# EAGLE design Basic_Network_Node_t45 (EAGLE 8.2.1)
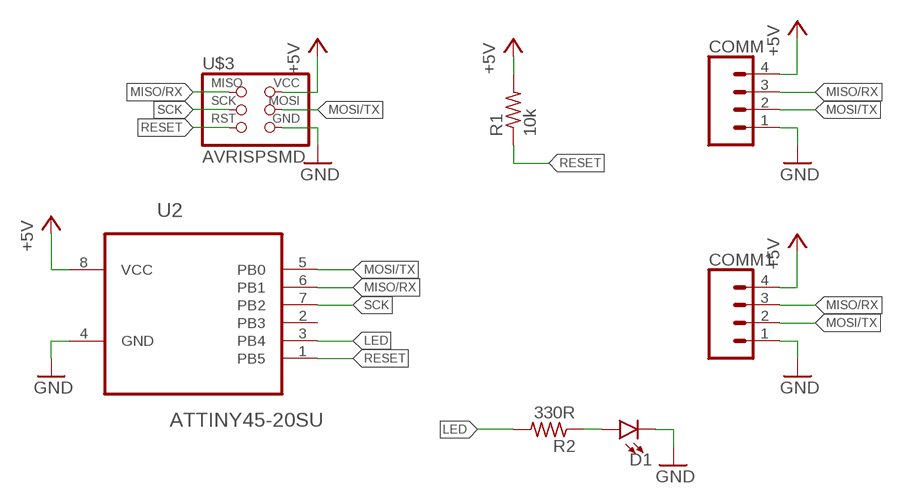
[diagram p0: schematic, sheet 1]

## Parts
COMM  CONN_04SMD_RA_FEMALE  [1X04_SMD_RA_FEMALE]
COMM1  CONN_04SMD_RA_FEMALE  [1X04_SMD_RA_FEMALE]
D1  LED1206  [LED-1206]
R1  10k  R-US_R1206  [R1206]
R2  330R  R-US_R1206  [R1206]
U2  ATTINY45-20SU  [SOIC127P798X216-8N]
U$3  AVRISPSMD  [2X03SMD]

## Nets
+5V: COMM1.4 COMM.4 R1.2 U2.8(VCC) U$3.2(VCC)
GND: COMM1.1 COMM.1 D1.C U2.4(GND) U$3.6(GND)
LED: R2.2 U2.3(PB4)
MISO/RX: COMM1.3 COMM.3 U2.6(PB1) U$3.1(MISO)
MOSI/TX: COMM1.2 COMM.2 U2.5(PB0) U$3.4(MOSI)
N$4: D1.A R2.1
RESET: R1.1 U2.1(PB5) U$3.5(RST)
SCK: U2.7(PB2) U$3.3(SCK)
Unconnected: U2.2(PB3)

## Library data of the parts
COMM COMM1 = SparkFun-Connectors:CONN_04: Multi connection point. Often used as Generic Header-pin footprint for 0.1 inch spaced/style header connections On any of the 0.1 inch spaced packages, you can populate with these: Break Away Headers - Straight (PRT-00116) Break Away Male Headers - Right Angle (PRT-00553) Female Headers (PRT-00115)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
D1 = SparkFun-LED:LED: LED (Generic)
R1 R2 = rcl:R-US_: RESISTOR, American symbol
U2 = Atmel_By_element14_Batch_1-00:ATTINY45-20SU: 8-bit Microcontroller with 4 Bytes In-System Programmable Flash; MPN: ATTINY45-20SU; OC_FARNELL: 1288353; OC_NEWARK: 23M5073; PACKAGE: SOIC-8; SUPPLIER: Atmel
U$3 = fab:AVRISP

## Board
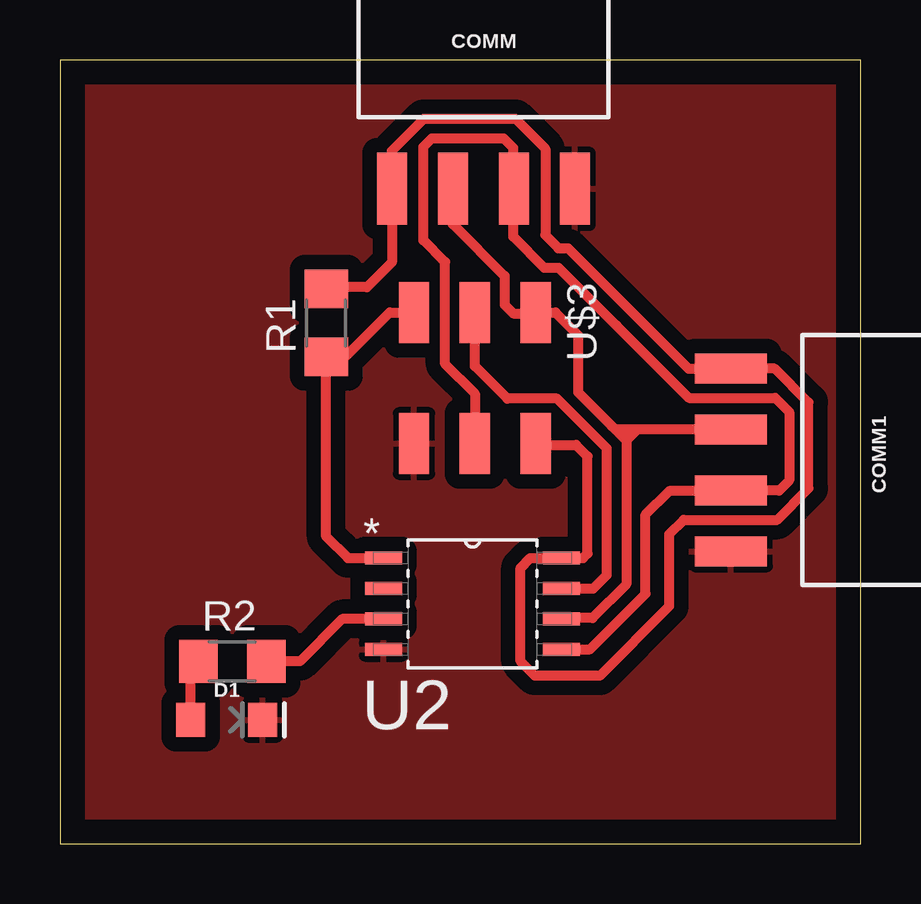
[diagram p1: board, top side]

Size 33.39 x 32.67 mm. Coordinates in mm from the lower left corner, seen from the top.
Outline: 0,0 33.39,0 33.39,32.67 0,32.67 0,0
Copper layers (1*16): Top 0.035mm / dielectric 1.5mm / Bottom 0.035mm
Design rules "default *": minimum track width 6mil, minimum drill 0.35mm, track to track 0.4mm, track to pad 0.4mm, pad to pad 0.4mm, via to via 0.4mm, smd to smd 6mil, copper to edge 40mil, drill to drill 6mil, minimum pad ring 10mil, minimum via ring 8mil, stop-mask expansion 4mil, vias tented up to drill 0mil, thermal gap 10mil

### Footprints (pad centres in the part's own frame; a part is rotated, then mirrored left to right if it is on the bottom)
1X04_SMD_RA_FEMALE = smd 1.25 x 3: 1 -3.81,7.225; 2 -1.27,7.225; 3 1.27,7.225; 4 3.81,7.225
LED-1206 = smd 1.2 x 1.4: A -1.5,0; C 1.5,0
R1206 = smd 1.6 x 1.803: 1 -1.422,0; 2 1.422,0
SOIC127P798X216-8N = smd 1.549 x 0.533: 1 -3.708,1.905; 2 -3.708,0.635; 3 -3.708,-0.635; 4 -3.708,-1.905; 5 3.708,-1.905; 6 3.708,-0.635; 7 3.708,0.635; 8 3.708,1.905
2X03SMD = smd 2.54 x 1.27: 1 -2.54,2.54; 2 2.92,2.54; 3 -2.54,0; 4 2.92,0; 5 -2.54,-2.54; 6 2.92,-2.54

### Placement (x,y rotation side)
COMM  17.65,34.53 180 top
COMM1  35.2,16 90 top
D1  6.95,5.16 0 top
R1  11.1,21.71 90 top
R2  7.19,7.6 0 top
U2  17.2,10 0 top
U$3  17.3,19.6 270 top

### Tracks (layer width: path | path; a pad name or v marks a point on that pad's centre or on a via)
+5V
  Top 0.406: U$3.2 19.9,16.62 21.52,16.62 21.99,16.14 21.99,12.09 21.8,11.9 U2.8 19.6,11.9 19.2,11.5 19.2,7.6 19.8,7 22.5,7 25.4,9.9 25.4,12.9 26,13.5 29.9,13.5 31.21,14.81 31.21,18.39 29.8,19.8 COMM1.4 | R1.2 11.03,23.2 12.8,23.2 13.84,24.24 COMM.4 | 13.9,26.96 COMM.4 | COMM1.4 | COMM1.4 26.2,19.8 21.18,24.82 20.78,24.82 20.23,25.37 20.23,28.97 18.99,30.21 15.17,30.21 13.84,28.88 COMM.4
GND
  pour Top (isolate 0.61): 0,32.6 33.2,32.6 33.2,0 0,0
LED
  Top 0.406: U2.3 11.77,9.37 10,7.6 R2.2
MISO/RX
  Top 0.406: 23.21,17.21 23.61,16.81 | 23.21,17.21 23.01,17.41 21.6,18.82 21.6,21.2 20.66,22.14 U$3.1 | 19.98,22 U$3.1 | U2.6 20.94,9.4 22.2,9.4 23.61,10.81 23.61,16.81 | COMM.3 16.38,25.82 18.54,23.66 18.54,22.46 18.9,22.1 19.8,22.1 U$3.1 | COMM1.3 24.06,17.27 | 24.06,17.27 23.61,16.81 | 24.06,17.27 23.27,17.27 23.21,17.21
MOSI/TX
  Top 0.406: U2.5 22.1,8.1 24.41,10.41 24.41,13.71 25.4,14.7 27.95,14.7 COMM1.2 29.98,14.72 30.4,15.14 30.4,18 29.82,18.58 26.23,18.58 23.21,21.6 23.2,21.6 20.79,24.01 20.19,24.01 18.9,25.3 18.9,27.32 | U$3.4 17.3,18.76 16.06,20 16.06,24.25 15.15,25.16 15.15,29.05 15.51,29.41 18.49,29.41 18.9,29 18.9,27.32 | COMM.2 19,26.98 | 18.9,26.89 COMM.2 | 18.9,27.32 COMM.2
N$4
  Top 0.406: D1.A 5.45,7.28 R2.1
RESET
  Top 0.406: U2.1 12,11.9 11.1,12.8 R1.1 11.89,20.29 13.74,22.14 U$3.5
SCK
  Top 0.406: U$3.3 17.3,19.9 18.65,18.55 20.73,18.55 22.8,16.48 22.8,11.2 22.23,10.63 U2.7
